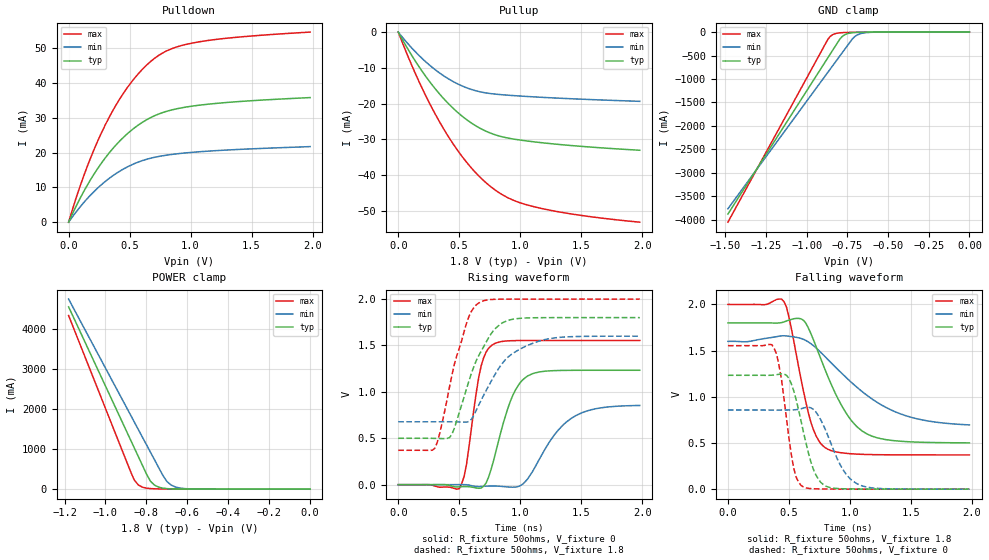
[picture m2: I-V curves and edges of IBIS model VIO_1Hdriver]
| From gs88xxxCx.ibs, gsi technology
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|  signals   DQA1-DQA9, DQB1-DQB9, DQC1-DQC9, DQD1-DQD9
[Model]   VIO_1Hdriver
Model_type   I/O
Polarity   Non-Inverting
Vinl  =   0.75v
Vinh  =   1.75v
Vmeas =   1.25v
Cref  =   0.0pF
Rref  =   50
Vref  =   1.25v
|  variable   typ   min   max
C_comp   3.0pF   2.5pF   3.5pF
|  variable   typ   min   max
[Temperature Range]   50   0   100
|  variable   typ   min   max
[Voltage Range]   1.8   1.6   2.0
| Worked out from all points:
|   slope of the pulldown table from 0 to 0.27 V, typ, clamps not added: 15.9 ohm
|   slope of the pullup table from 0 to 0.27 V, typ, clamps not added: 18.7 ohm
|   GND clamp passes 1 mA (typ) near -0.61 V on its own axis
|   POWER clamp passes 1 mA (typ) near -0.59 V on its own axis
|   rising waveform, R_fixture 50ohms, V_fixture 0: 20-80 % time 169ps typ, 273ps min, 104ps max; typ from 0 V to 1.23 V
|   rising waveform, R_fixture 50ohms, V_fixture 1.8: 20-80 % time 226ps typ, 279ps min, 180ps max; typ from 0.5 V to 1.8 V
|   falling waveform, R_fixture 50ohms, V_fixture 1.8: 20-80 % time 278ps typ, 500ps min, 158ps max; typ from 1.8 V to 0.501 V
|   falling waveform, R_fixture 50ohms, V_fixture 0: 20-80 % time 137ps typ, 179ps min, 96.6ps max; typ from 1.23 V to 0 V
[Pulldown]
| voltage   typ   min   max
0V        -278.2pA   -874.6pA   -161.2pA
80mV      5.892mA    3.774mA    8.899mA
160mV     11.04mA    7.053mA    16.68mA
240mV     15.52mA    9.871mA    23.46mA
320mV     19.37mA    12.26mA    29.32mA
400mV     22.64mA    14.25mA    34.36mA
500mV     26mA       16.22mA    39.6mA
600mV     28.62mA    17.66mA    43.8mA
700mV     30.54mA    18.63mA    47.01mA
840mV     32.24mA    19.46mA    49.82mA
1.06V     33.6mA     20.23mA    51.82mA
1.98V     35.84mA    21.75mA    54.68mA
[Pullup]
| voltage (VDDQ-Vout)   typ   min   max
0V        191.8pA    794.2pA    89.01pA
80mV      -4.802mA   -3.277mA   -6.819mA
180mV     -10.18mA   -6.867mA   -14.56mA
280mV     -14.87mA   -9.905mA   -21.45mA
380mV     -18.89mA   -12.4mA    -27.52mA
560mV     -24.48mA   -15.57mA   -36.39mA
660mV     -26.69mA   -16.61mA   -40.22mA
760mV     -28.3mA    -17.21mA   -43.28mA
920mV     -29.76mA   -17.7mA    -46.67mA
1.12V     -30.72mA   -18.13mA   -48.9mA
1.48V     -31.9mA    -18.73mA   -51.17mA
1.98V     -33.04mA   -19.37mA   -53.16mA
[GND Clamp]
| voltage   typ   min   max
-1.485V   -3.884A    -3.771A    -4.056A
-885mV    -626.9mA   -926.9mA   -247.2mA
-870mV    -545.6mA   -856mA     -153.5mA
-855mV    -464.4mA   -785mA     -89.11mA
-825mV    -301.9mA   -643.2mA   -32.88mA
-795mV    -141.5mA   -501.4mA   -15.38mA
-780mV    -86.61mA   -430.5mA   -11.65mA
-750mV    -32.85mA   -288.8mA   -7.734mA
-705mV    -8.727mA   -95.28mA   -4.834mA
-660mV    -2.907mA   -24.97mA   -2.925mA
-555mV    -316.7uA   -1.176mA   -484.9uA
0V        -278.2pA   -874.6pA   -161.2pA
[POWER Clamp]
| voltage (VDDQ-Vout)   typ   min   max
-1.18V    4.545A     4.74A      4.328A
-880mV    1.258A     1.875A     474.1mA
-860mV    1.039A     1.684A     234.3mA
-840mV    820.4mA    1.493A     107.4mA
-820mV    601.5mA    1.302A     50.64mA
-780mV    197.3mA    920.5mA    14.28mA
-760mV    99.71mA    729.7mA    9.034mA
-720mV    26.23mA    348.2mA    4.898mA
-700mV    13.96mA    192.6mA    3.916mA
-660mV    4.495mA    57.55mA    2.579mA
-560mV    510.5uA    2.941mA    648.3uA
0V        209pA      794.1pA    88.9pA
[Ramp]
| voltage   typ   min   max
dV/dt_r   1.15/174p   0.98/260p   1.35/124p
dV/dt_f   1.18/177p   1.01/270p   1.36/124p
R_load  =   50ohms
[Rising Waveform]
C_fixture =   0.0pF
R_fixture =   50ohms
V_fixture =   0
| Time   V(typ)   V(min)   V(max)
0s        2.823nV    12.42nV    1.162nV
500ps     -24.11mV   538.6uV    -42.81mV
560ps     -20.81mV   -833.6uV   222.4mV
680ps     -35.85mV   -19.33mV   1.282V
780ps     252.6mV    -14.58mV   1.514V
920ps     902.1mV    -26.51mV   1.551V
1.06ns    1.171V     60.12mV    1.554V
1.28ns    1.229V     537.1mV    1.554V
1.42ns    1.232V     715.8mV    1.554V
1.98ns    1.233V     853.5mV    1.554V
[Rising Waveform]
C_fixture =   0.0pF
R_fixture =   50ohms
V_fixture =   1.8
V_fixture_min =  1.6
V_fixture_max =  2.0
| Time   V(typ)   V(min)   V(max)
0s        499.9mV    677.7mV    370.5mV
300ps     498.6mV    677.8mV    392.8mV
340ps     497.2mV    677.7mV    553mV
440ps     543.3mV    677.8mV    1.179V
580ps     1.12V      680.6mV    1.815V
660ps     1.392V     858.5mV    1.958V
840ps     1.732V     1.285V     1.999V
1.06ns    1.797V     1.5V       2V
1.32ns    1.8V       1.587V     2V
1.98ns    1.8V       1.6V       2V
[Falling Waveform]
C_fixture =   0.0pF
R_fixture =   50ohms
V_fixture =   1.8
V_fixture_min =  1.6
V_fixture_max =  2.0
| Time   V(typ)   V(min)   V(max)
0s        1.8V       1.6V       2V
460ps     1.811V     1.66V      2.03V
500ps     1.83V      1.656V     1.865V
600ps     1.844V     1.631V     1.187V
680ps     1.685V     1.575V     726.1mV
800ps     1.282V     1.43V      446.4mV
980ps     802mV      1.196V     386.5mV
1.14ns    597.8mV    1.016V     375.5mV
1.5ns     512.1mV    778.7mV    371mV
1.98ns    501.4mV    695.7mV    370.6mV
[Falling Waveform]
C_fixture =   0.0pF
R_fixture =   50ohms
V_fixture =   0
| Time   V(typ)   V(min)   V(max)
0s        1.233V     856.8mV    1.554V
380ps     1.236V     856.4mV    1.521V
440ps     1.248V     856.7mV    1.182V
540ps     1.064V     858.2mV    225.4mV
620ps     614.2mV    878.2mV    22.52mV
700ps     218.3mV    864.5mV    4.717mV
760ps     74.79mV    753.6mV    2.619mV
940ps     4.51mV     218.9mV    686.4uV
1.06ns    2.006mV    57.57mV    278uV
1.98ns    16.58uV    329.6uV    887.2nV
